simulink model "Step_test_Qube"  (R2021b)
settings: Solver=ode1  StartTime=0.0  StopTime=2.5  FixedStep=0.002  RelTol=1e-3  AbsTol=1e-6  EnableMultiTasking=on
undefined symbols (not defined in the file or in its folder): HIL
libraries: quarc_library x3

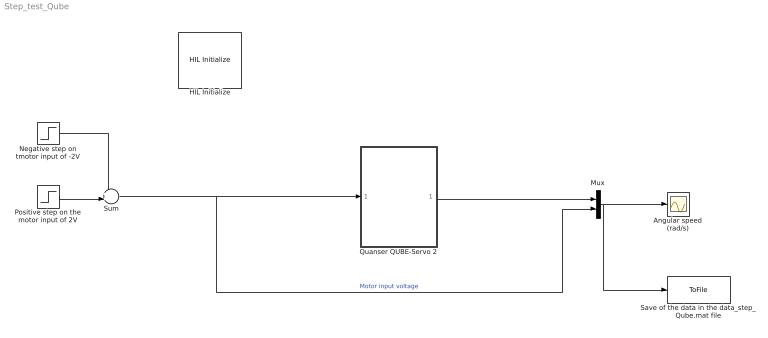
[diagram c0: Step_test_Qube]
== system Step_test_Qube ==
  Angular speed (rad/s) : Scope
  HIL Initialize : quarc_library/Data Acquisition/Generic/Configuration/HIL Initialize  Priority=-99  object_name=HIL-1  board_type=qube_servo2_usb  board_number=0  board_options=""  exclusive=off  active=off  hardware_clocks=[0]  clock_modes=[]  initial_clock_frequencies=[]  set_clock_params_at_start=off  set_clock_params_at_switch_in=off  set_clock_frequencies_at_start=off  set_clock_frequencies_at_switch_in=off  analog_input_channels=[0]  analog_input_configurations=[]  analog_input_maximums=3  analog_input_minimums=-3  set_analog_input_params_at_start=off  set_analog_input_params_at_switch_in=off  analog_output_channels=[0]  analog_output_maximums=15  analog_output_minimums=-15  initial_analog_outputs=[0]  final_analog_outputs=[0]  watchdog_analog_outputs=0  set_analog_output_params_at_start=off  set_analog_output_params_at_switch_in=off  set_analog_outputs_at_start=on  set_analog_outputs_at_switch_in=off  set_analog_outputs_at_terminate=on  set_analog_outputs_at_switch_out=off  set_analog_outputs_on_watchdog=on  digital_input_channels=[]  digital_output_channels=[0]  digital_output_configuration=[]  initial_digital_outputs=[1]  final_digital_outputs=[0]  watchdog_digital_outputs=[0]  set_digital_output_params_at_start=off  set_digital_output_params_at_switch_in=off  set_digital_outputs_at_start=on  set_digital_outputs_at_switch_in=off  set_digital_outputs_at_terminate=on  set_digital_outputs_at_switch_out=off  set_digital_outputs_on_watchdog=on  encoder_channels=[0:1]  quadrature=[4]  encoder_filter_frequency=[]  initial_encoder_counts=[0]  set_encoder_params_at_start=off  set_encoder_params_at_switch_in=off  set_encoder_counts_at_start=on  set_encoder_counts_at_switch_in=off  pwm_channels=[]  pwm_modes=[]  pwm_frequency=[]  pwm_configuration=[]  pwm_alignment=[]  pwm_polarity=[]  pwm_leading_deadband=[]  pwm_trailing_deadband=[]  initial_pwm_outputs=[]  final_pwm_outputs=[]  watchdog_pwm_outputs=[]  set_pwm_params_at_start=off  set_pwm_params_at_switch_in=off  set_pwm_outputs_at_start=off  set_pwm_outputs_at_switch_in=off  set_pwm_outputs_at_terminate=off  set_pwm_outputs_at_switch_out=off  set_pwm_outputs_on_watchdog=off  other_output_channels=[11000:11002]  initial_other_outputs=[0 1 0]  final_other_outputs=[1 0 0]  watchdog_other_outputs=[0 0 1]  set_other_outputs_at_start=on  set_other_outputs_at_switch_in=off  set_other_outputs_at_terminate=on  set_other_outputs_at_switch_out=off  set_other_outputs_on_watchdog=on
  Mux : Mux  Inputs=2
  Negative step on tmotor input of -2V : Step  Time=2.5  After=-2  SampleTime=0
  Positive step on the motor input of 2V : Step  After=2  SampleTime=0
  Quanser QUBE-Servo 2 : Subsystem
  Save of the data in the data_step_Qube.mat file : ToFile  Filename=data_step_Qube.mat  MatrixName=data_step
  Sum : Sum  Inputs=++|
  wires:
  Quanser QUBE-Servo 2/1(Angular velocity (rad/s)) -> Mux/1
  Mux/1 -> Save of the data in the data_step_Qube.mat file/1, Angular speed (rad/s)/1
  Positive step on the motor input of 2V/1 -> Sum/2
  Sum/1 -> Quanser QUBE-Servo 2/1(In1), Mux/2  "Motor input voltage"
  Negative step on tmotor input of -2V/1 -> Sum/1

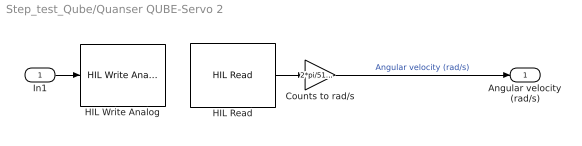
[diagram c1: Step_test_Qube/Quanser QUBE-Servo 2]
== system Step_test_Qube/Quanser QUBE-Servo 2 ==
  In1 : Inport
  Counts to rad/s : Gain  Gain=2*pi/512/4
  HIL Read : quarc_library/Data Acquisition/Generic/Immediate I//O/HIL Read  object_name=HIL-1  analog_channels=[]  encoder_channels=[]  digital_channels=[]  other_channels=[14000]  sample_time=qc_get_step_size  active=on  vector_output=off  data_type_mode=Inherit via back propagation  encoder_data_type=double  digital_data_type=boolean
  HIL Write Analog : quarc_library/Data Acquisition/Generic/Immediate I//O/HIL Write Analog  object_name=HIL-1  channels=0  sample_time=-1  active=off  vector_input=off
  Angular velocity (rad/s) : Outport
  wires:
  In1/1 -> HIL Write Analog/1
  Counts to rad/s/1 -> Angular velocity (rad/s)/1  "Angular velocity (rad/s)"
  HIL Read/1 -> Counts to rad/s/1
